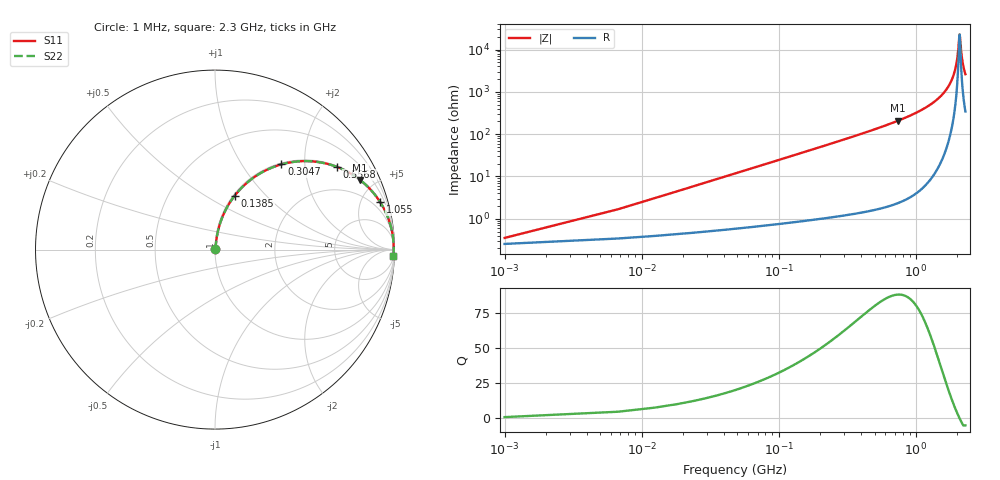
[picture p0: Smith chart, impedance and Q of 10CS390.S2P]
! Coilcraft 1008CS-390 Chip Inductor
! 02 July 2002
# MHZ S MA R 50
!Freq  MagS11  AngS11  MagS21  AngS21  MagS12  AngS12  MagS22  AngS22
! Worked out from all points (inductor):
!   403 points, 1 MHz to 2.3 GHz, reference 50 ohm
!   read as one part in series: L = 39 nH near 12.46 MHz
!   highest Q = 88.5 at 740.2 MHz (marker M1), where L = 44.6 nH
!   self-resonance near 2.087 GHz
!   S11 on the Smith chart (normalised r, x): 1 MHz: 1.01, +0.00; 138.5 MHz: 1.02, +0.68; 304.7 MHz: 1.02, +1.53; 556.8 MHz: 1.04, +2.94; 1.055 GHz: 1.09, +6.95; 2.3 GHz: 8, -52
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1  0.003528 43.7  0.9975 -0.1  0.9975 -0.1  0.003528 43.7
18.19  0.04455 81.9  0.9947 -2.5  0.9947 -2.5  0.04455 81.9
35.38  0.08611 81.6  0.9911 -4.9  0.9911 -4.9  0.08611 81.6
75.49  0.1811 77.5  0.9769 -10.4  0.9769 -10.4  0.1811 77.5
138.52  0.3203 69.9  0.9393 -18.7  0.9393 -18.7  0.3203 69.9
213.01  0.4629 61.3  0.8775 -27.6  0.8775 -27.6  0.4629 61.3
304.69  0.602 52.1  0.789 -37.0  0.789 -37.0  0.602 52.1
384.91  0.6938 45.3  0.7105 -43.9  0.7105 -43.9  0.6938 45.3
556.81  0.8221 34.0  0.5596 -55.3  0.5596 -55.3  0.8221 34.0
740.17  0.8969 25.6  0.4323 -63.7  0.4323 -63.7  0.8969 25.6
768.82  0.905 24.5  0.4152 -64.8  0.4152 -64.8  0.905 24.5
1055.32  0.9577 16.0  0.2757 -73.3  0.2757 -73.3  0.9577 16.0
1152.73  0.9678 13.8  0.2382 -75.4  0.2382 -75.4  0.9678 13.8
1536.64  0.9893 6.9  0.1205 -81.5  0.1205 -81.5  0.9893 6.9
1765.84  0.9942 3.8  0.06553 -83.0  0.06553 -83.0  0.9942 3.8
1920.55  0.9955 1.9  0.03282 -81.2  0.03282 -81.2  0.9955 1.9
2006.5  0.9957 0.9  0.01607 -74.0  0.01607 -74.0  0.9957 0.9
2086.72  0.9956 0.0  0.004383 -3.4  0.004383 -3.4  0.9956 0.0
2098.18  0.9956 -0.1  0.004785 22.9  0.004785 22.9  0.9956 -0.1
2144.02  0.9954 -0.6  0.01123 65.6  0.01123 65.6  0.9954 -0.6
2184.13  0.9952 -1.0  0.01809 74.1  0.01809 74.1  0.9952 -1.0
2300  0.9943 -2.2  0.03793 80.3  0.03793 80.3  0.9943 -2.2
